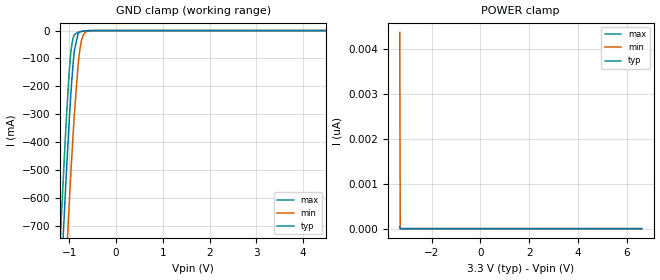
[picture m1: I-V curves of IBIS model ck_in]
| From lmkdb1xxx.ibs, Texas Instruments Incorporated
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| Model1
|IBIS Model File - Generated by SIMDE
| http://www.iometh.com/Product/SIMDE
[Model]   ck_in
Model_type   Input
Vinl = 0.66
Vinh = 2.64
|   typ   min   max
C_comp   3pF   2.5pF   3.5pF
[Voltage Range]   3.3   3.135   3.465
[Temperature Range]   27   125   -40
[Power Clamp Reference]   3.3   3.135   3.465
[GND Clamp Reference]   0   0   0
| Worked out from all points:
|   GND clamp passes 1 mA (typ) near -0.68 V on its own axis
[GND Clamp]
|   Voltage   I(typ)   I(min)   I(max)
-3.3V     -9.039A    -9.284A    -8.888A
-1.191V   -935.5mA   -1.251A    -732mA
-1.162V   -831.2mA   -1.146A    -628.1mA
-1.092V   -595.1mA   -906.9mA   -396mA
-1.023V   -374.9mA   -677.1mA   -191.4mA
-973.5mV  -234.8mA   -521.5mA   -82.42mA
-894.3mV  -70.11mA   -296.5mA   -14.46mA
-815.1mV  -10.89mA   -123.3mA   -6.064mA
-765.6mV  -4.002mA   -55.99mA   -4.283mA
-716.1mV  -1.883mA   -21.3mA    -2.535mA
-557.7mV  -94.7uA    -711uA     -73.04uA
6.6V      0A         0A         0A
[POWER Clamp]
|   Voltage   I(typ)   I(min)   I(max)
-3.3V     45.09pA    4.378nA    27.16pA
-3.28V    0A         0A         0A
-3.27V    0A         0A         0A
6.6V      0A         0A         0A
